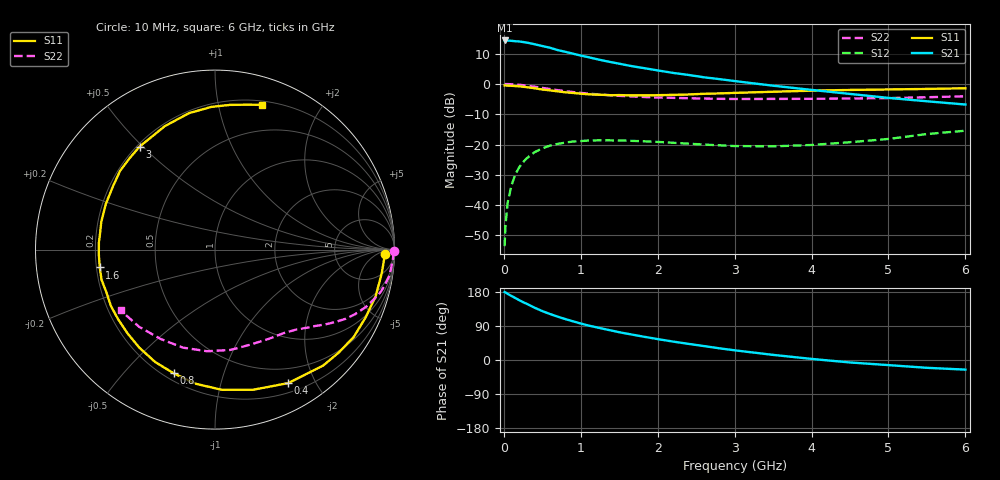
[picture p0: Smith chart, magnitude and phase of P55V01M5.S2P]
! SIEMENS Small Signal Semiconductors
! BFP183
! Si NPN RF Bipolar Junction Transistor in SOT143
! VCE = 5 V  IC = 1.5 mA
! Common Emitter S-Parameters:  March  1996
# GHz  S  MA  R  50
!  f  S11  S21  S12  S22
! GHz  MAG  ANG  MAG  ANG  MAG  ANG  MAG  ANG
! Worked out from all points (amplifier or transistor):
!   36 points, 10 MHz to 6 GHz, reference 50 ohm
!   highest |S21| = 14.3 dB at 10 MHz (marker M1)
!   |S21| within 3 dB of that: start of sweep to 676.7 MHz
!   unconditionally stable (mu >= 1): 2.288 GHz to 5.939 GHz
!   at 250 MHz: K = 0.11, MSG = 19.8 dB, |S12| = -25.8 dB
!   at 1.4 GHz: K = 0.60, MSG = 12.9 dB, |S12| = -18.6 dB
!   at 6 GHz: K = 0.99, MSG = 4.3 dB, |S12| = -15.4 dB
!   S11 on the Smith chart (normalised r, x): 10 MHz: 29, -14; 400 MHz: 0.31, -1.64; 800 MHz: 0.24, -0.69; 1.6 GHz: 0.21, -0.07; 3 GHz: 0.21, +0.49; 6 GHz: 0.24, +1.35
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0.01  0.9452 -1.5  5.217 179.2  0.0021 85.7  0.9993 -0.6
0.02  0.9438 -3.3  5.203 178.3  0.0044 85.9  0.9934 -1.1
0.05  0.9382 -8.2  5.192 174.4  0.0111 87.0  0.9932 -2.8
0.1  0.932 -16.1  5.145 168.9  0.0213 79.8  0.987 -5.8
0.2  0.9134 -32.2  5.02 157.9  0.0422 71.2  0.9687 -11.4
0.25  0.8971 -39.7  4.915 152.6  0.0511 67.0  0.9537 -14.2
0.4  0.8481 -61.3  4.518 138.0  0.0747 55.1  0.8997 -20.8
0.5  0.8093 -74.8  4.217 129.0  0.0863 47.9  0.8599 -24.7
0.6  0.7821 -87.2  3.956 121.4  0.0959 42.0  0.8235 -27.9
0.7  0.7552 -98.2  3.617 114.4  0.1024 36.7  0.7891 -30.5
0.8  0.7268 -108.4  3.388 107.9  0.1077 31.9  0.7595 -32.8
1  0.69 -127.7  2.936 96.3  0.114 24.4  0.7105 -36.6
1.1  0.6748 -136.2  2.761 90.9  0.1162 21.1  0.6913 -38.3
1.3  0.6597 -151.5  2.418 81.9  0.1172 15.6  0.6607 -41.5
1.6  0.6498 -171.2  2.036 69.5  0.116 9.7  0.6278 -45.7
1.9  0.6469 171.4  1.756 58.7  0.1117 6.0  0.6032 -50.4
2.2  0.6594 157.1  1.52 48.6  0.1068 3.9  0.5889 -55.2
3  0.7113 126.2  1.115 25.6  0.0943 6.0  0.5642 -70.5
3.5  0.7425 112.1  0.935 13.5  0.0932 11.9  0.5656 -81.2
4.5  0.7954 91.4  0.684 -6.5  0.1092 22.9  0.5747 -108.1
5.5  0.8269 77.5  0.517 -20.6  0.1488 25.7  0.6032 -134.5
6  0.848 72.0  0.457 -25.4  0.1691 22.7  0.6254 -147.2
